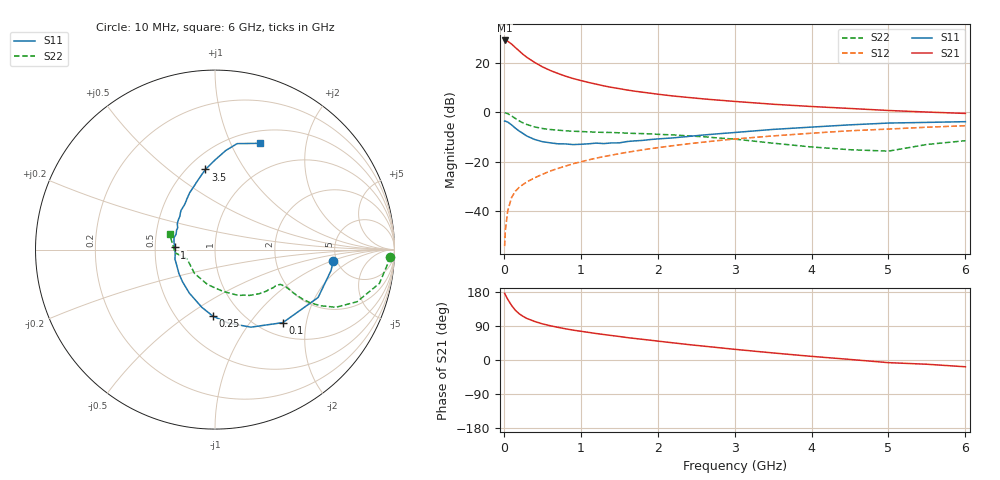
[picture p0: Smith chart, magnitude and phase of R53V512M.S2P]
! SIEMENS Small Signal Semiconductors
! BFR183
! Si NPN RF Bipolar Junction Transistor in SOT23
! VCE = 3.5 V  IC = 12 mA
! Common Emitter S-Parameters:  May  1996
# GHz  S  MA  R  50
!  f  S11  S21  S12  S22
! GHz  MAG  ANG  MAG  ANG  MAG  ANG  MAG  ANG
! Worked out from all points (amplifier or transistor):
!   36 points, 10 MHz to 6 GHz, reference 50 ohm
!   highest |S21| = 28.9 dB at 10 MHz (marker M1)
!   |S21| within 3 dB of that: start of sweep to 155.5 MHz
!   unconditionally stable (mu >= 1): 718.7 MHz to 2.461 GHz
!   at 250 MHz: K = 0.68, MSG = 26.2 dB, |S12| = -29.1 dB
!   at 1.4 GHz: K = 1.05, MAG = 12.3 dB, |S12| = -17.3 dB
!   at 6 GHz: K = 0.89, MSG = 2.5 dB, |S12| = -5.5 dB
!   S11 on the Smith chart (normalised r, x): 10 MHz: 4.68, -1.02; 100 MHz: 1.25, -1.47; 250 MHz: 0.74, -0.64; 1 GHz: 0.63, +0.02; 3.5 GHz: 0.61, +0.68; 6 GHz: 0.64, +1.30
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0.01  0.6616 -5.3  27.8 175.9  0.002 84.5  0.9748 -2.3
0.02  0.6573 -10.1  27.66 171.7  0.0042 85.5  0.9657 -4.7
0.05  0.6334 -24.9  26.85 160.4  0.0102 79.6  0.9353 -11.6
0.1  0.5554 -47.1  23.57 144.2  0.019 71.7  0.8423 -20.2
0.15  0.476 -65.2  20.03 131.1  0.0256 66.7  0.7462 -25.5
0.2  0.416 -79.7  17.09 122.0  0.0307 65.0  0.6664 -28.0
0.25  0.3711 -91.8  14.59 115.1  0.035 63.8  0.6061 -29.2
0.3  0.3299 -102.8  12.7 109.6  0.0394 64.6  0.5641 -29.5
0.4  0.2818 -120.4  10.05 101.8  0.0476 65.4  0.5047 -29.0
0.5  0.2547 -135.3  8.202 95.4  0.0559 65.7  0.4694 -28.2
0.6  0.2413 -146.4  6.954 90.6  0.0649 66.9  0.4478 -27.8
0.7  0.2308 -157.1  6.044 86.3  0.0733 67.2  0.4339 -27.8
0.8  0.2293 -166.8  5.318 82.4  0.0819 67.0  0.4221 -27.9
1  0.2254 176.9  4.33 75.8  0.1 67.2  0.4074 -28.6
1.1  0.2307 171.1  3.972 72.9  0.1092 66.8  0.4014 -29.7
1.3  0.233 158.6  3.386 67.2  0.1276 65.7  0.3916 -31.4
1.6  0.2559 145.2  2.795 59.2  0.1553 63.6  0.3777 -35.4
2.2  0.3034 123.7  2.116 45.3  0.2116 58.4  0.3483 -44.9
3.5  0.4496 96.9  1.444 18.6  0.3323 43.1  0.2373 -79.1
4.5  0.5553 83.8  1.187 1.5  0.4226 30.7  0.1752 -130.5
5.5  0.622 71.9  1.005 -11.2  0.4975 18.9  0.2235 -175.6
6  0.6433 67.0  0.943 -17.9  0.5332 11.3  0.2663 161.3
